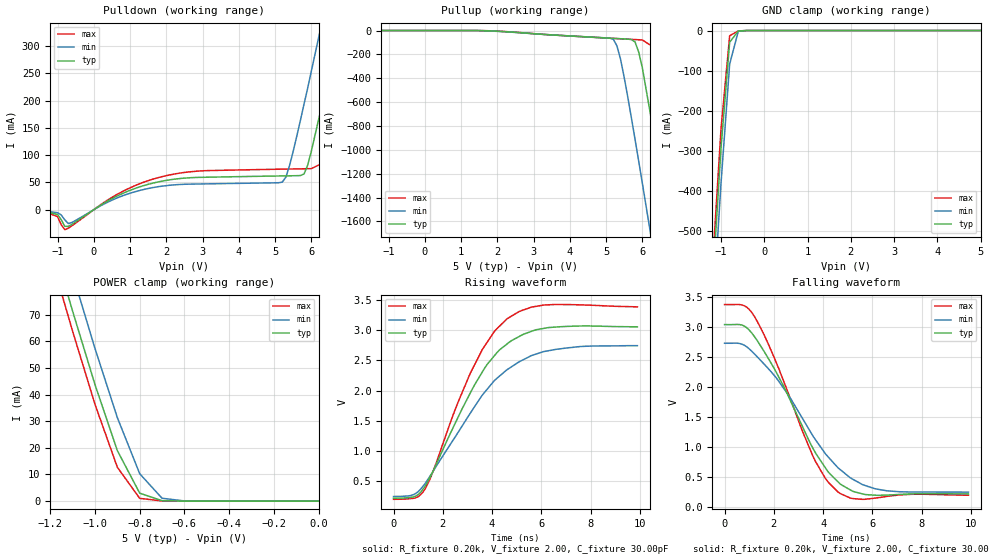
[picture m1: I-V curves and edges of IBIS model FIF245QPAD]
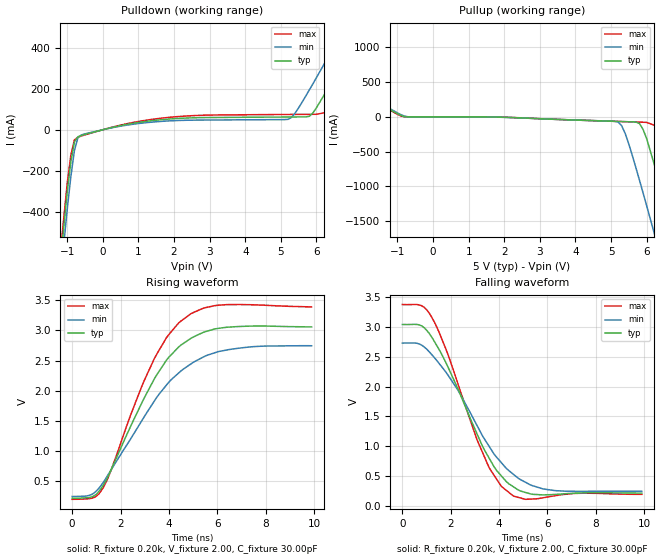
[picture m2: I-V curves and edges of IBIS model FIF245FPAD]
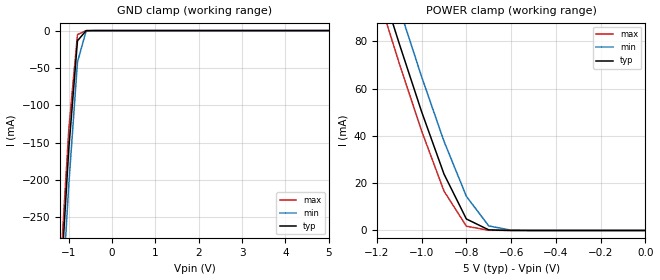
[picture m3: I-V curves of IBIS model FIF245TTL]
| IBIS file idt72235.ibs created by s2ibis2 version 1.1
| North Carolina State University Electronics Research Laboratory  1995
[IBIS ver]   2.1
[File name]   idt72235.ibs
[File Rev]   1.0
[Date]   08/26/97
[Source]   Integrated Device Technology, Inc.
[Notes]   1. Temperatures: typ=25C, min=70C, max=0C 2. Cemos8_5v
   process. 3. Ramp rates based on 50 ohm load.
[Copyright]   Copyright 1997, Integrated Device Technology, Inc.
|   Component idt72235
[Component]   idt72235
[Manufacturer]   Integrated Device Technology
[Package]
| variable   typ   min   max
R_pkg   0.75   0.60   0.90
L_pkg   8.10nH   8.30nH   9.90nH
C_pkg   0.53pF   0.46pF   0.60pF
[Pin]  signal_name   model_name   R_pin   L_pin   C_pin
1   D15   FIF245TTL
2   D14   FIF245TTL
3   D13   FIF245TTL
4   D12   FIF245TTL
5   D11   FIF245TTL
6   D10   FIF245TTL
7   D9   FIF245TTL
8   D8   FIF245TTL
9   D7   FIF245TTL
10   D6   FIF245TTL
11   D5   FIF245TTL
12   D4   FIF245TTL
13   D3   FIF245TTL
14   D2   FIF245TTL
15   D1   FIF245TTL
16   D0   FIF245TTL
17   PAEL   FIF245FPAD
18   FLB   FIF245TTL
19   WCLK   FIF245TTL
20   WENL   FIF245TTL
21   WXIL   FIF245TTL
22   VCC   POWER
23   PAFL   FIF245FPAD
24   RXIL   FIF245TTL
25   FFL   FIF245FPAD
26   WXOLHF   FIF245FPAD
27   RXOL   FIF245FPAD
28   Q0   FIF245QPAD
29   Q1   FIF245QPAD
30   GND   GND
31   Q2   FIF245QPAD
32   Q3   FIF245QPAD
33   VCC   POWER
34   Q4   FIF245QPAD
35   GND   GND
36   Q5   FIF245QPAD
37   Q6   FIF245QPAD
38   Q7   FIF245QPAD
39   Q8   FIF245QPAD
40   GND   GND
41   Q9   FIF245QPAD
42   Q10   FIF245QPAD
43   VCC   POWER
44   Q11   FIF245QPAD
45   Q12   FIF245QPAD
46   GND   GND
47   Q13   FIF245QPAD
48   Q14   FIF245QPAD
49   VCC   POWER
50   Q15   FIF245QPAD
51   GND   GND
52   Q16   FIF245QPAD
53   Q17   FIF245QPAD
54   EFL   FIF245FPAD
55   GND   GND
56   VCC   POWER
57   RSL   FIF245TTL
58   OEL   FIF245TTL
59   LDL   FIF245TTL
60   RENL   FIF245TTL
61   RCLK   FIF245TTL
62   GND   GND
63   D17   FIF245TTL
64   D16   FIF245TTL
| Models and submodels in the file (3): FIF245QPAD (3-state), FIF245FPAD (Output), FIF245TTL (Input)
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| FIN  FIN   dummy_model
| QIN  QIN   dummy_model
| QOEL QOEL   dummy_model
|   Model FIF245QPAD
[Model]   FIF245QPAD
Model_type   3-state
Polarity   Non-Inverting
Enable   Active-Low
Vmeas =  1.500V
C_comp   3.00pF   NA   NA
[Temperature Range]   25.00   70.00   0.000
[Voltage Range]   5.00V   4.50V   5.50V
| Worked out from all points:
|   slope of the pulldown table from 0 to 0.75 V, typ, clamps not added: 26.4 ohm
|   GND clamp passes 1 mA (typ) near -0.58 V on its own axis
|   POWER clamp passes 1 mA (typ) near -0.73 V on its own axis
|   rising waveform, R_fixture 0.20k, V_fixture 2.00, C_fixture 30.00pF: 20-80 % time 2.17ns typ, 2.59ns min, 1.95ns max; typ from 0.212 V to 3.06 V
|   falling waveform, R_fixture 0.20k, V_fixture 2.00, C_fixture 30.00pF: 20-80 % time 2.11ns typ, 2.47ns min, 1.85ns max; typ from 3.04 V to 0.213 V
[Pulldown]
| voltage   I(typ)   I(min)   I(max)
-5V       0A         0A         0A
-1.4V     -3mA       -2mA       -2.6mA
-800mV    -30.42mA   -18.6mA    -36.69mA
1.7V      49.86mA    41.4mA     57.4mA
5.2V      62.01mA    50.61mA    74.43mA
5.4V      62.22mA    81.07mA    74.66mA
5.8V      65.63mA    194mA      75.11mA
6V        107mA      254mA      75.33mA
6.4V      223mA      376mA      88.46mA
6.8V      345mA      500mA      198mA
7.2V      469mA      624mA      320mA
10V       1.346A     1.502A     1.195A
[Pullup]
| voltage   I(typ)   I(min)   I(max)
-5V       0A         0A         0A
1.5V      -479uA     -1.046mA   -164uA
5.2V      -65.7mA    -73.36mA   -65.97mA
5.3V      -67.33mA   -129mA     -67.59mA
5.4V      -68.96mA   -242mA     -69.22mA
5.8V      -96.18mA   -914mA     -75.69mA
6V        -312mA     -1.279A    -78.93mA
6.4V      -1.008A    -2.023A    -157mA
6.8V      -1.75A     -2.776A    -778mA
7.2V      -2.503A    -3.534A    -1.516A
7.6V      -3.262A    -4.295A    -2.268A
10V       -7.849A    -8.885A    -6.849A
[GND_clamp]
| voltage   I(typ)   I(min)   I(max)
-5V       -7.849A    -7.926A    -7.807A
-1.2V     -640mA     -729mA     -591mA
-1V       -293mA     -381mA     -246mA
-800mV    -29.29mA   -83.51mA   -12.91mA
-600mV    -1.086mA   -1.828mA   -995uA
-400mV    -11.7nA    -1.657uA   -4.457nA
5V        50nA       1.239uA    50nA
[POWER_clamp]
| voltage   I(typ)   I(min)   I(max)
-5V       1.28A      1.292A     1.273A
-1.2V     100mA      114mA      92.56mA
-1.1V     71.31mA    85.16mA    63.76mA
-1V       43.75mA    57.31mA    36.34mA
-900mV    18.98mA    31.36mA    12.72mA
-800mV    2.991mA    10.3mA     1.049mA
-700mV    169uA      1.084mA    64.47uA
-600mV    6.517uA    77.91uA    260nA
0V        50nA       45nA       55nA
[Ramp]
| variable   typ   min   max
dV/dt_r   1.00/1.23n   0.85/1.56n   1.15/1.10n
dV/dt_f   1.67/2.34n   1.36/2.85n   1.96/2.01n
R_load = 50.00
[Rising Waveform]
R_fixture = 0.20k
V_fixture = 2.00
C_fixture = 30.00pF
R_dut = 0.75
L_dut = 8.10nH
C_dut = 0.53pF
| time   V(typ)   V(min)   V(max)
0s        212mV      240mV      193mV
900ps     246mV      290mV      218mV
1.3ns     421mV      464mV      378mV
3.1ns     1.947V     1.614V     2.272V
3.8ns     2.434V     2.021V     2.802V
4.6ns     2.771V     2.344V     3.19V
5.3ns     2.94V      2.52V      3.343V
6.1ns     3.033V     2.648V     3.421V
7.6ns     3.073V     2.732V     3.424V
9.9ns     3.059V     2.746V     3.391V
[Falling Waveform]
R_fixture = 0.20k
V_fixture = 2.00
C_fixture = 30.00pF
R_dut = 0.75
L_dut = 8.10nH
C_dut = 0.53pF
| time   V(typ)   V(min)   V(max)
0s        3.045V     2.733V     3.38V
800ps     3.021V     2.7V       3.36V
1.2ns     2.852V     2.56V      3.19V
2.2ns     2.168V     2.097V     2.31V
3.6ns     967mV      1.174V     833mV
4.1ns     647mV      881mV      468mV
4.6ns     419mV      653mV      248mV
5.2ns     258mV      460mV      136mV
6.2ns     190mV      293mV      148mV
9.9ns     213mV      243mV      192mV
|   Model FIF245FPAD
[Model]   FIF245FPAD
Model_type   Output
Vmeas =  1.500V
C_comp   3.00pF   NA   NA
[Temperature Range]   25.00   70.00   0.000
[Voltage Range]   5.00V   4.50V   5.50V
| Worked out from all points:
|   slope of the pulldown table from 0 to 0.75 V, typ, clamps not added: 26.4 ohm
|   rising waveform, R_fixture 0.20k, V_fixture 2.00, C_fixture 30.00pF: 20-80 % time 2.15ns typ, 2.57ns min, 1.96ns max; typ from 0.212 V to 3.06 V
|   falling waveform, R_fixture 0.20k, V_fixture 2.00, C_fixture 30.00pF: 20-80 % time 1.91ns typ, 2.24ns min, 1.69ns max; typ from 3.04 V to 0.212 V
[Pulldown]
| voltage   I(typ)   I(min)   I(max)
-5V       -7.849A    -7.926A    -7.807A
-1.4V     -1.006A    -1.093A    -958mA
-1V       -302mA     -386mA     -259mA
-800mV    -59.72mA   -102mA     -49.6mA
-600mV    -27.75mA   -25.16mA   -30.34mA
5.2V      62.01mA    50.61mA    74.43mA
5.8V      65.63mA    194mA      75.11mA
6.4V      223mA      376mA      88.46mA
6.8V      345mA      500mA      198mA
7.2V      469mA      624mA      320mA
8V        718mA      874mA      568mA
10V       1.346A     1.502A     1.195A
[Pullup]
| voltage   I(typ)   I(min)   I(max)
-5V       1.28A      1.292A     1.273A
-1.4V     160mA      173mA      152mA
-800mV    2.991mA    10.3mA     1.049mA
5.2V      -65.7mA    -73.36mA   -65.97mA
5.4V      -68.96mA   -242mA     -69.22mA
5.8V      -96.18mA   -914mA     -75.69mA
6V        -312mA     -1.279A    -78.93mA
6.4V      -1.008A    -2.023A    -157mA
6.8V      -1.75A     -2.776A    -778mA
7.2V      -2.503A    -3.534A    -1.516A
7.6V      -3.262A    -4.295A    -2.268A
10V       -7.849A    -8.885A    -6.849A
[Ramp]
| variable   typ   min   max
dV/dt_r   1.00/1.24n   0.85/1.51n   1.15/1.07n
dV/dt_f   1.67/1.85n   1.36/2.26n   1.96/1.61n
R_load = 50.00
[Rising Waveform]
R_fixture = 0.20k
V_fixture = 2.00
C_fixture = 30.00pF
R_dut = 0.75
L_dut = 8.10nH
C_dut = 0.53pF
| time   V(typ)   V(min)   V(max)
0s        212mV      240mV      193mV
800ps     231mV      272mV      210mV
1.3ns     435mV      482mV      396mV
2.9ns     1.812V     1.512V     2.092V
3.4ns     2.196V     1.827V     2.533V
3.9ns     2.506V     2.092V     2.88V
4.5ns     2.757V     2.327V     3.156V
5.4ns     2.964V     2.553V     3.365V
6.1ns     3.037V     2.653V     3.42V
9.9ns     3.058V     2.745V     3.391V
[Falling Waveform]
R_fixture = 0.20k
V_fixture = 2.00
C_fixture = 30.00pF
R_dut = 0.75
L_dut = 8.10nH
C_dut = 0.53pF
| time   V(typ)   V(min)   V(max)
0s        3.045V     2.733V     3.38V
800ps     3.022V     2.698V     3.36V
1.2ns     2.843V     2.547V     3.178V
1.8ns     2.406V     2.246V     2.634V
2.3ns     1.963V     1.942V     2.048V
3.1ns     1.197V     1.339V     1.097V
3.6ns     791mV      991mV      631mV
4.5ns     343mV      558mV      192mV
6ns       184mV      271mV      146mV
9.9ns     212mV      242mV      191mV
|   Model FIF245TTL
[Model]   FIF245TTL
Model_type   Input
Vinl =  0.000V
Vinh =  3.000V
Vmeas =  1.500V
C_comp   3.00pF   NA   NA
[Temperature Range]   25.00   70.00   0.000
[Voltage Range]   5.00V   4.50V   5.50V
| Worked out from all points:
|   GND clamp passes 1 mA (typ) near -0.61 V on its own axis
|   POWER clamp passes 1 mA (typ) near -0.72 V on its own axis
[GND_clamp]
| voltage   I(typ)   I(min)   I(max)
-5V       -4.391A    -4.433A    -4.368A
-1.2V     -352mA     -401mA     -325mA
-1V       -158mA     -206mA     -132mA
-800mV    -13.65mA   -42.02mA   -5.426mA
-600mV    -95.68uA   -488uA     -19.8uA
5V        50nA       2.529uA    50nA
[POWER_clamp]
| voltage   I(typ)   I(min)   I(max)
-5V       1.33A      1.343A     1.323A
-1.2V     109mA      124mA      101mA
-1.1V     79.07mA    94.22mA    70.74mA
-1V       50.25mA    65.05mA    42.12mA
-900mV    23.87mA    37.74mA    16.67mA
-800mV    4.863mA    14.45mA    1.814mA
-700mV    253uA      1.929mA    79.02uA
-600mV    7.842uA    115uA      476nA
0V        50nA       45nA       55nA
